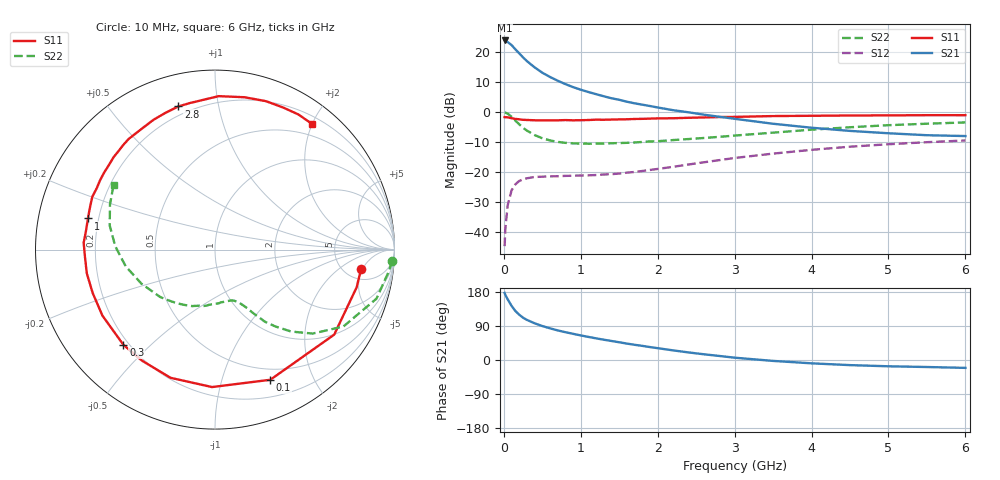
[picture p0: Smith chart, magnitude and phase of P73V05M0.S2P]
! SIEMENS Small Signal Semiconductors
! BFP196
! Si NPN RF Bipolar Junction Transistor in SOT143
! VCE = 3 V  IC = 5 mA
! Common Emitter S-Parameters:  May  1996
# GHz  S  MA  R  50
!  f  S11  S21  S12  S22
! GHz  MAG  ANG  MAG  ANG  MAG  ANG  MAG  ANG
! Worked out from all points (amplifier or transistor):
!   36 points, 10 MHz to 6 GHz, reference 50 ohm
!   highest |S21| = 23.9 dB at 10 MHz (marker M1)
!   |S21| within 3 dB of that: start of sweep to 150.9 MHz
!   unconditionally stable (mu >= 1): 1.119 GHz to 3.197 GHz
!   at 250 MHz: K = 0.26, MSG = 20.4 dB, |S12| = -22.5 dB
!   at 1.4 GHz: K = 1.16, MAG = 10.3 dB, |S12| = -20.8 dB
!   at 6 GHz: K = 0.99, MSG = 0.7 dB, |S12| = -9.5 dB
!   S11 on the Smith chart (normalised r, x): 10 MHz: 7.02, -4.68; 100 MHz: 0.38, -1.44; 300 MHz: 0.18, -0.41; 1 GHz: 0.16, +0.12; 2.8 GHz: 0.15, +0.76; 6 GHz: 0.31, +1.99
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0.01  0.8211 -7.6  15.73 176.9  0.0057 86.5  0.9884 -3.7
0.02  0.8167 -14.9  15.46 171.5  0.0114 81.9  0.9768 -7.0
0.05  0.8158 -35.5  14.79 160.1  0.0276 72.1  0.9404 -16.9
0.1  0.788 -67.0  13.2 143.0  0.0487 57.6  0.834 -30.9
0.15  0.7661 -91.2  11.17 129.3  0.0618 46.2  0.7175 -40.7
0.2  0.756 -109.1  9.595 119.5  0.0702 39.0  0.6232 -47.1
0.25  0.7404 -123.5  8.188 111.6  0.0747 33.5  0.5438 -51.9
0.3  0.736 -133.9  7.107 105.8  0.0779 29.9  0.4884 -55.3
0.4  0.7271 -149.6  5.583 96.9  0.082 25.1  0.4112 -59.1
0.5  0.7231 -160.4  4.544 89.6  0.0828 22.7  0.3641 -61.8
0.6  0.7264 -169.5  3.856 83.6  0.0838 21.6  0.3346 -64.5
0.7  0.7258 -177.2  3.337 78.1  0.0843 21.2  0.3165 -66.9
0.8  0.7328 177.0  2.928 73.4  0.0854 21.3  0.3048 -69.3
1  0.7289 166.2  2.359 64.9  0.0866 22.8  0.2961 -74.2
1.1  0.7349 161.6  2.158 60.9  0.0872 24.1  0.2949 -77.2
1.6  0.7559 141.5  1.486 43.3  0.0967 32.2  0.3052 -92.9
2.2  0.7865 121.8  1.073 25.4  0.1211 38.9  0.3394 -112.0
2.8  0.8232 104.4  0.833 10.7  0.1566 39.5  0.384 -132.6
3.5  0.8552 88.6  0.636 -2.4  0.2014 34.3  0.4515 -155.1
4.5  0.8743 71.1  0.483 -13.5  0.263 23.0  0.5559 178.1
5.5  0.8848 58.3  0.409 -18.5  0.3127 10.4  0.6371 156.7
6  0.8844 52.5  0.396 -20.8  0.3339 3.7  0.6696 147.6
